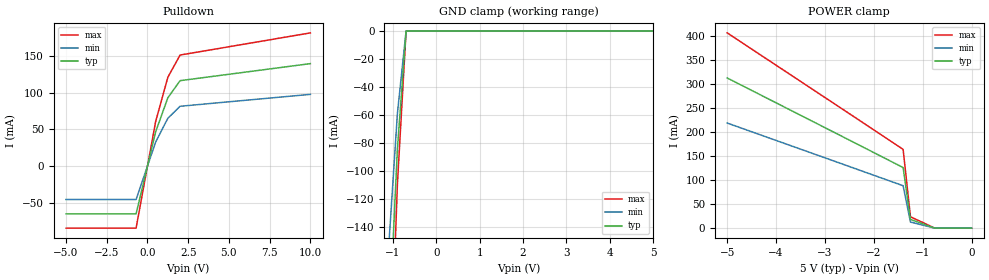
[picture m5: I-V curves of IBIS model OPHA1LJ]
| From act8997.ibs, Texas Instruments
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[Model]   OPHA1LJ
| 16-mA n-channel open-drain CMOS/TTL output buffer with 0.125 di/dt
| OP (97318 ALEY)
| BP (97318 ALEY)
Model_type   Open_drain
Polarity   Non-Inverting
| Signals   DCO (open-drain)
| variable   typ   min   max
C_comp   15pF   NA   NA
| variable   typ   min   max
[Voltage range]   5.0V   4.5V   5.5V
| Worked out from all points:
|   slope of the pulldown table from 0 to 0.75 V, typ, clamps not added: 12.1 ohm
|   GND clamp passes 1 mA (typ) near -0.70 V on its own axis
[pulldown]
|   50C:5V:   100C:4.5V:weak  0C:5.5V:strong
| Voltage   I(typ)   I(min)   I(max)
-5V       -65.3mA    -45.7mA    -84.9mA
-900mV    -65.3mA    -45.7mA    -84.9mA
-700mV    -65.3mA    -45.7mA    -84.9mA
-500mV    -46.7mA    -32.7mA    -60.7mA
0V        0A         0A         0A
500mV     46.7mA     32.7mA     60.7mA
1.25V     93.3mA     65.3mA     121.3mA
2V        116.7mA    81.7mA     151.7mA
10V       140mA      98mA       182mA
[power_clamp]
|   50C:5V:   100C:4.5V:weak  0C:5.5V:strong
| Voltage   I(typ)   I(min)   I(max)
-5V       312.2mA    218.5mA    405.9mA
-2.75V    196mA      137.2mA    254.8mA
-1.4V     126mA      88.2mA     163.8mA
-1.25V    18.2mA     12.7mA     23.7mA
-750mV    0A         0A         0A
0V        0A         0A         0A
[gnd_clamp]
|   50C:5V:   100C:4.5V:weak  0C:5.5V:strong
| Voltage   I(typ)   I(min)   I(max)
-5V       -2.8A      -2A        -3.6A
-900mV    -84mA      -58.8mA    -109.2mA
-700mV    0A         0A         0A
0V        0A         0A         0A
5V        0A         0A         0A
[ramp]
| variable   typ   min   max
dV/dt_r   2.3/2.25e-9   1.9/3.375e-9   2.7/1.5e-9
dV/dt_f   2.3/3e-9   1.9/4.5e-9   2.7/2e-9
